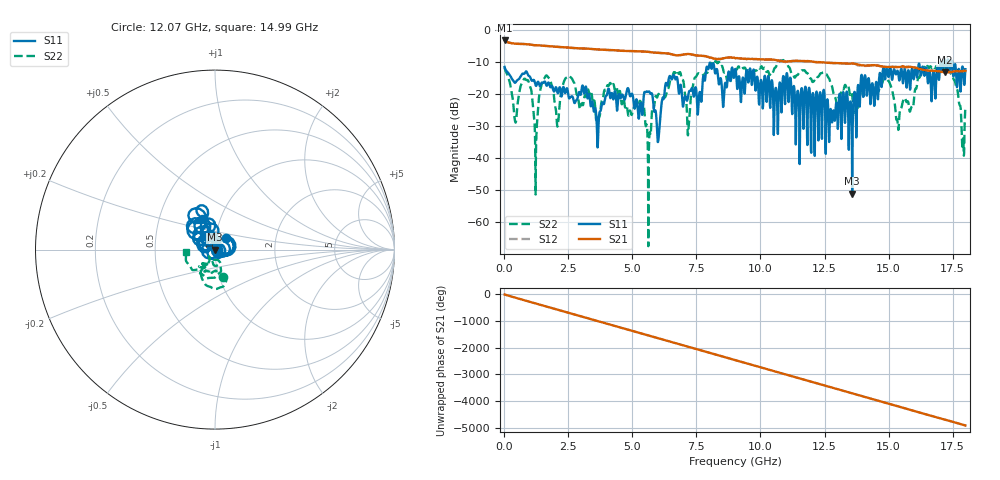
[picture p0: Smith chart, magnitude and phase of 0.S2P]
!Agilent Technologies,E5071C,MY46316741,A.11.02
!Date: Thu Sep 29 15:39:46 2022
!Data & Calibration Information:
!Freq	S11:SOLT2(ON)	S21:SOLT2(ON)	S12:SOLT2(ON)	S22:SOLT2(ON)
!PortZ  Port1:50+j0  Port2:50+j0
!Above PortZ is port z conversion or system Z0 setting when saving the data.
!When reading, reference impedance value at option line is always used.
# Hz S dB R 50
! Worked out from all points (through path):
!   1800 points, 10 MHz to 18 GHz, reference 50 ohm
!   highest |S21| = -3.23 dB at 10 MHz (marker M1); lowest = -13.2 dB at 17.19 GHz (marker M2)
!   group delay of S21, straight-line fit = 758 ps
!   lowest |S11| = -51.0 dB at 13.58 GHz (marker M3), VSWR 1.01, Z = 49.7 - j0.0611 ohm
!   |S11| at or under -10 dB: start of sweep to 17.04 GHz; 17.05 GHz to 17.15 GHz (98.82 MHz wide, 0.578 % of centre); 17.48 GHz to end of sweep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
!   |S22| runs from -67.4 to -9.3 dB; largest |S21 - S12| = 0.027
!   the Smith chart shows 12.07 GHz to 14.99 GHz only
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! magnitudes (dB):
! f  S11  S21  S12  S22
! 10 MHz  -11.5  -3.2  -3.2  -11.6
! 430 MHz  -16.4  -4.2  -4.2  -28.7
! 950 MHz  -14.2  -4.5  -4.5  -16.1
! 1.22 GHz  -17.2  -4.7  -4.7  -51.3
! 1.6 GHz  -16.3  -4.9  -4.9  -14.5
! 2.06 GHz  -19.0  -5.2  -5.2  -29.7
! 2.47 GHz  -18.7  -5.5  -5.5  -14.5
! 3.01 GHz  -18.9  -5.7  -5.7  -22.9
! 3.66 GHz  -33.2  -6.1  -6.1  -27.1
! 4.2 GHz  -19.6  -6.2  -6.3  -17.5
! 5.64 GHz  -19.1  -6.8  -6.8  -37.8
! 6.01 GHz  -34.4  -7.1  -7.1  -20.0
! 6.52 GHz  -15.2  -7.5  -7.5  -15.1
! 7.18 GHz  -20.2  -7.5  -7.5  -31.7
! 7.52 GHz  -22.1  -7.9  -8.0  -14.0
! 9.01 GHz  -12.2  -8.7  -8.8  -12.4
! 12.01 GHz  -22.5  -9.8  -9.8  -15.9
! 13.58 GHz  -51.0  -10.4  -10.4  -20.4
! 15.01 GHz  -14.3  -11.5  -11.5  -16.0
! 15.36 GHz  -12.8  -11.5  -11.5  -29.4
! 17.19 GHz  -9.0  -13.2  -13.2  -11.8
! 18 GHz  -12.2  -12.7  -12.8  -24.4
